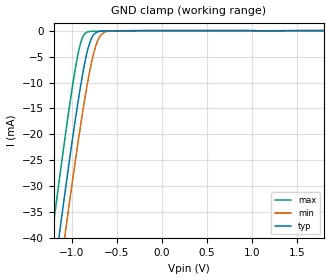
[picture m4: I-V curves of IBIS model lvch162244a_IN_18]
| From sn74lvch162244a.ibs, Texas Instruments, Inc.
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[Model]   lvch162244a_IN_18
Model_type  Input
Vinl=0.5775
Vinh=1.2675
| variable   typ   min   max
C_comp   3.30pF   2.57pF   4.39pF
[Temperature Range]   40   100   -40
| Ambient temperature   25   85   -40
[Voltage range]   1.8   1.65   1.95
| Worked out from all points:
|   GND clamp passes 1 mA (typ) near -0.76 V on its own axis
[GND Clamp]
| lvch162244a_IN_18
|   Voltage   I(typ)   I(min)   I(max)
-5.5V     -656.7mA   -663.4mA   -648.4mA
-1.21V    -49.13mA   -57.37mA   -38.57mA
-1.135V   -39.24mA   -47.49mA   -28.66mA
-1.075V   -31.5mA    -39.72mA   -20.98mA
-1.055V   -28.97mA   -37.17mA   -18.48mA
-955mV    -16.8mA    -24.75mA   -7.051mA
-885mV    -9.203mA   -16.62mA   -1.639mA
-835mV    -4.749mA   -11.31mA   -352.1uA
-785mV    -1.753mA   -6.69mA    -146.1uA
-715mV    -275.1uA   -2.171mA   -107.4uA
-650mV    -80.87uA   -478.9uA   -91.3uA
1.8V      5.126pA    37.8nA     -54.32pA
